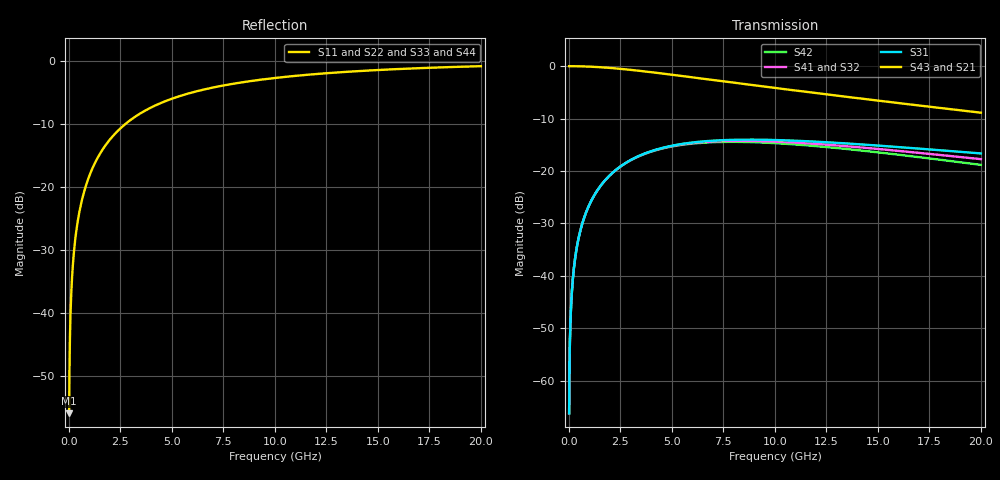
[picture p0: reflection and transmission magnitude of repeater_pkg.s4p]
! Libra (TM) Ver. 3.500.103.3
! Fri Dec 18 11:27:40 2009
! Number of ports is 4
# Hz	S	RI	R	50.000000
! SCATTERING PARAMETERS  :
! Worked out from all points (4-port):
!   2000 points, 10 MHz to 20 GHz, reference 50 ohm
!   strongest paths, dB at 10 MHz, 5.01 GHz, 10.01 GHz, 15.01 GHz, 20 GHz:
!     S43: 0.0, -1.6, -4.2, -6.6, -8.9
!     S21: 0.0, -1.6, -4.2, -6.6, -8.9
!     S31: -66.2, -15.2, -14.1, -15.2, -16.7
!     S41: -66.2, -15.2, -14.4, -15.8, -17.7
!     S32: -66.2, -15.2, -14.4, -15.8, -17.7
!     S42: -66.2, -15.3, -14.7, -16.4, -18.8
!   lowest |S11| = -55.9 dB at 10 MHz (marker M1), VSWR 1.00, Z = 50.1 + j0.126 ohm
!   |S11| at or under -10 dB: start of sweep to 2.734 GHz
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1e7  0.001 0.00125  0.999 -0.00152  1.23e-06 0.000489  -1.36e-06 -0.000489
     0.999 -0.00152  0.001 0.00125  -1.36e-06 -0.000489  1.49e-06 0.000489
     1.23e-06 0.000489  -1.36e-06 -0.000489  0.001 0.00125  0.999 -0.00152
     -1.36e-06 -0.000489  1.49e-06 0.000489  0.999 -0.00152  0.001 0.00125
2.1e8  0.00178 0.0263  0.998 -0.0319  0.00054 0.0102  -0.000598 -0.0102
       0.998 -0.0319  0.00211 0.0263  -0.000598 -0.0102  0.000655 0.0102
       0.00054 0.0102  -0.000598 -0.0102  0.00178 0.0263  0.998 -0.0319
       -0.000598 -0.0102  0.000655 0.0102  0.998 -0.0319  0.00211 0.0263
6.5e8  0.00842 0.0807  0.9899 -0.0978  0.00511 0.0311  -0.00565 -0.031
       0.9899 -0.0978  0.0115 0.0803  -0.00565 -0.031  0.00618 0.0309
       0.00511 0.0311  -0.00565 -0.031  0.00842 0.0807  0.9899 -0.0978
       -0.00565 -0.031  0.00618 0.0309  0.9899 -0.0978  0.0115 0.0803
1.58e9  0.0426 0.1877  0.9478 -0.2277  0.0281 0.0685  -0.031 -0.0672
        0.9478 -0.2277  0.06 0.1829  -0.031 -0.0672  0.0337 0.0658
        0.0281 0.0685  -0.031 -0.0672  0.0426 0.1877  0.9478 -0.2277
        -0.031 -0.0672  0.0337 0.0658  0.9478 -0.2277  0.06 0.1829
3.1e9  0.1385 0.323  0.8291 -0.3916  0.0871 0.0972  -0.0945 -0.0894
       0.8291 -0.3916  0.1951 0.2927  -0.0945 -0.0894  0.1012 0.081
       0.0871 0.0972  -0.0945 -0.0894  0.1385 0.323  0.8291 -0.3916
       -0.0945 -0.0894  0.1012 0.081  0.8291 -0.3916  0.1951 0.2927
1.08e10  0.5978 0.4669  0.247 -0.5381  0.1893 -0.0475  -0.1621 0.0943
         0.247 -0.5381  0.7617 0.03  -0.1621 0.0943  0.1245 -0.1302
         0.1893 -0.0475  -0.1621 0.0943  0.5978 0.4669  0.247 -0.5381
         -0.1621 0.0943  0.1245 -0.1302  0.247 -0.5381  0.7617 0.03
2e10  0.8326 0.372  -0.0244 -0.359  0.1009 -0.107  -0.0341 0.1252
      -0.0244 -0.359  0.7243 -0.5619  -0.0341 0.1252  -0.0255 -0.1115
      0.1009 -0.107  -0.0341 0.1252  0.8326 0.372  -0.0244 -0.359
      -0.0341 0.1252  -0.0255 -0.1115  -0.0244 -0.359  0.7243 -0.5619
